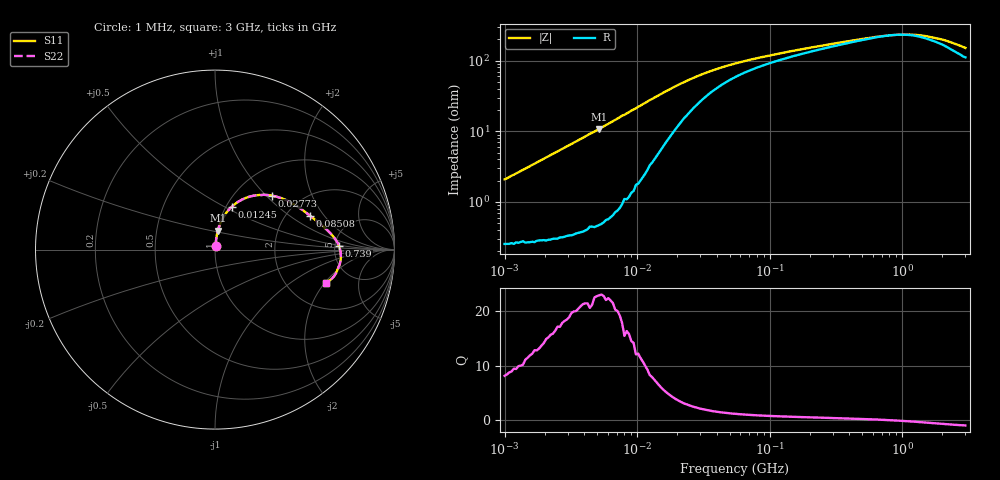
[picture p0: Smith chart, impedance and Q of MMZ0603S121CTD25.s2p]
! S-parameter Generated by TDK Corporation
! Copyright(C) 2018 TDK Corporation.
! All Rights Reserved.
! TDK P/N: MMZ0603S121CTD25 (Chip Bead)
! Property: |Z|=120¶ at 100MHz
! Size(LxWxT): 0.6x0.3x0.3mm, 0.024x0.012x0.012inches
! Model Type: s2p (Touchstone File Format Version 1.0)
! Frequency: DC=Yes Start=1MHz Stop=3000MHz 202points Log-sweep
! Model Generated on Aug. 6, 2018
! Port Assignments:
!  1 ---@@@--- 2
! Applicable Conditions:
!  Temperature = 25 degC
!  DC Bias Current = 0 A
!  Small Signal Operation
! Terms and conditions regarding TDK Simulation Models
! (1)This simulation model is being provided solely for informational purposes. Please refer to the specifications of the products in terms of detailed characteristics of such products.
! (2)In no event shall TDK Corporation of any of its subsidiaries be liable for any loss or damage arising, directly or indirectly,
!  From any information contained in this simulation model, including, but not limited to loss or damages arising from any inaccuracies, omissions or errors in connection with such information.
! (3)Any and all copyrights on this simulation model are owned by TDK Corporation.
!  Duplication or redistribution of this simulation model without prior written permission from TDK Corporation is prohibited.
! (4)This simulation model is subject to any modification or change without any prior notice.
! (5)Neither TDK Corporation nor any of its subsidiaries shall make any warranty, express or implied,
!  Including but not limited to the correctness, implied warranties of merchantability and fitness for a particular purpose with respect to this simulation models.
! (6)The use of this simulation model shall be deemed to have consented to the terms and conditions hereof.
# Hz S MA R 50
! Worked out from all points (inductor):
!   201 points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, 1 MHz to 3 GHz, reference 50 ohm
!   read as one part in series: L = 328 nH near 1.041 MHz
!   highest Q = 22.7 at 5.162 MHz (marker M1), where L = 332 nH
!   self-resonance near 864.2 MHz
!   S11 on the Smith chart (normalised r, x): 1 MHz: 1.01, +0.04; 12.45 MHz: 1.07, +0.55; 27.73 MHz: 1.46, +1.08; 85.08 MHz: 2.66, +1.47; 739 MHz: 5.46, +0.38; 3 GHz: 3.21, -2.06
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1000000  0.02086 81.8  0.9972 -1.2  0.9972 -1.2  0.02086 81.8
2055611  0.0423 83.7  0.9963 -2.4  0.9963 -2.4  0.0423 83.7
3900413  0.0804 82.7  0.993 -4.6  0.993 -4.6  0.0804 82.7
5161903  0.1067 81.4  0.9896 -6.1  0.9896 -6.1  0.1067 81.4
7703107  0.1624 77.4  0.9776 -9.3  0.9776 -9.3  0.1624 77.4
8686058  0.1813 75.9  0.972 -10.4  0.972 -10.4  0.1813 75.9
1.061086e7  0.2203 72.3  0.9564 -12.7  0.9564 -12.7  0.2203 72.3
1.245355e7  0.2584 68.3  0.9356 -14.9  0.9356 -14.9  0.2584 68.3
1.461624e7  0.296 64.2  0.9109 -17.0  0.9109 -17.0  0.296 64.2
2.013356e7  0.3734 53.8  0.8359 -21.1  0.8359 -21.1  0.3734 53.8
2.773354e7  0.4381 43.3  0.7443 -23.8  0.7443 -23.8  0.4381 43.3
3.976269e7  0.4909 33.1  0.6471 -24.5  0.6471 -24.5  0.4909 33.1
5.477226e7  0.5249 26.3  0.5786 -23.7  0.5786 -23.7  0.5249 26.3
8.507507e7  0.5617 19.7  0.5077 -21.9  0.5077 -21.9  0.5617 19.7
2.136344e8  0.6251 11.0  0.4043 -17.1  0.4043 -17.1  0.6251 11.0
4.570858e8  0.6691 5.5  0.3401 -10.9  0.3401 -10.9  0.6691 5.5
7.38967e8  0.6916 1.5  0.3092 -3.4  0.3092 -3.4  0.6916 1.5
8.005644e8  0.6946 0.8  0.3056 -1.7  0.3056 -1.7  0.6946 0.8
1.10276e9  0.7021 -2.7  0.3004 6.2  0.3004 6.2  0.7021 -2.7
1.45942e9  0.7005 -6.2  0.313 14.0  0.313 14.0  0.7005 -6.2
2.177892e9  0.6831 -11.9  0.3602 23.0  0.3602 23.0  0.6831 -11.9
3e9  0.6445 -16.9  0.4264 26.0  0.4264 26.0  0.6445 -16.9
